TYPE "EN_Acknowledge"
VERSION : 0.1


  STRUCT
   OK : BYTE ;	//OK
   SERVICE_IS_NOT_SUPPORTED : BYTE  := B#16#1;	//Service is not supported | Check service ID in the request data
   DATA_LENGTH_INVALID : BYTE  := B#16#2;	//Data length invalid | Check data length in the request data
   OBJECT_INDEX_INVALID : BYTE  := B#16#3;	//Object index invalid | Check index and sub index of the object in the request d
   ACCESS_TYPE_INVALID : BYTE  := B#16#4;	//Access type invalid | Check access type of the object in the request data
   DATA_TYPE_INVALID : BYTE  := B#16#5;	//Data type invalid | Check data type of the object in the request data
   VALUE_INVALID : BYTE  := B#16#6;	//Value invalid | Check range of values of the object in the request data
   READ_TYPE_INVALID : BYTE  := B#16#7;	//Read type invalid | Check read type in the request data
   WRITE_TYPE_INVALID : BYTE  := B#16#8;	//Write type invalid | Check write type in the request data
   VALUES_INVALID : BYTE  := B#16#9;	//Values invalid | Check range of values of the object in the request data
  END_STRUCT ;
END_TYPE

